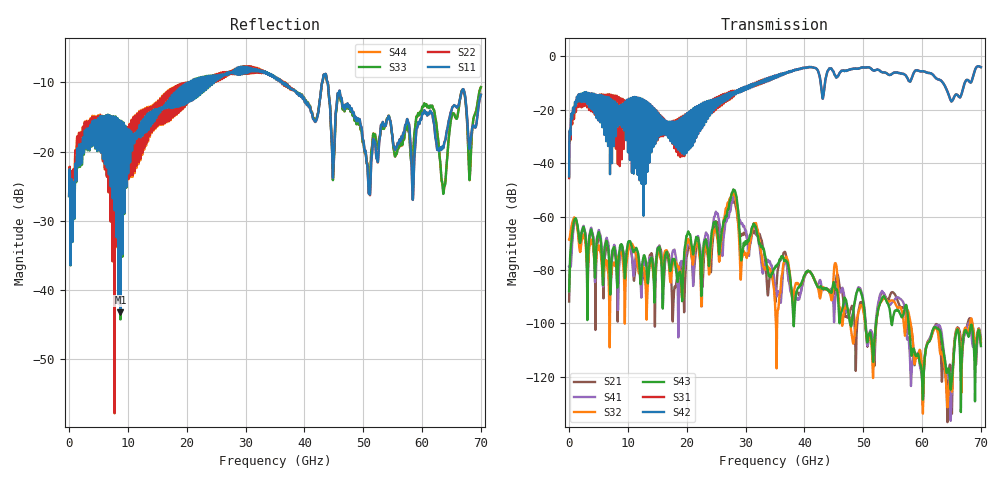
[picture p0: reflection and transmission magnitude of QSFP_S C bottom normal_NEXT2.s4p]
! AWR Design Environment (8415) Tue Jan 08 12:00:01 2019
! Document = 'QSFP Channel_S'
! nPorts: 4, nXvals: 7001
# HZ S DB R 50
!Freq DBS11 AngS11 DBS12 AngS12 DBS13 AngS13 DBS14 AngS14
!	DBS21 AngS21 DBS22 AngS22 DBS23 AngS23 DBS24 AngS24
!	DBS31 AngS31 DBS32 AngS32 DBS33 AngS33 DBS34 AngS34
!	DBS41 AngS41 DBS42 AngS42 DBS43 AngS43 DBS44 AngS44
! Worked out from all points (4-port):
!   7000 points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, 10 MHz to 70 GHz, reference 50 ohm
!   strongest paths, dB at 10 MHz, 17.51 GHz, 35.01 GHz, 52.51 GHz, 70 GHz:
!     S42: -44.9, -29.9, -7.3, -5.0, -4.0
!     S31: -45.6, -27.8, -7.4, -5.0, -4.0
!     S43: -88.0, -76.9, -79.1, -94.9, -108.5
!     S32: -68.7, -79.6, -92.6, -95.2, -106.9
!     S41: -78.7, -74.4, -85.9, -92.7, -107.5
!     S21: -91.8, -91.3, -91.2, -93.8, -105.6
!   lowest |S11| = -43.2 dB at 8.73 GHz (marker M1), VSWR 1.01, Z = 49.5 - j0.488 ohm
!   |S11| at or under -10 dB: start of sweep to 20.43 GHz; 36.44 GHz to 43.04 GHz (6.602 GHz wide, 16.6 % of centre); 43.96 GHz to end of sweep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
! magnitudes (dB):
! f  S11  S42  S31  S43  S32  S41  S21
! 10 MHz  -26.4  -44.9  -45.6  -88.0  -68.7  -78.7  -91.8
! 1.63 GHz  -20.1  -14.2  -15.6  -66.9  -69.1  -67.9  -67.3
! 8.73 GHz  -43.2  -21.2  -17.0  -70.6  -73.1  -72.3  -72.8
! 22.51 GHz  -10.0  -19.1  -19.6  -87.6  -91.6  -86.2  -78.4
! 27.87 GHz  -8.5  -13.6  -13.9  -50.2  -51.2  -53.1  -53.8
! 34.07 GHz  -8.8  -8.8  -8.9  -82.0  -79.4  -76.7  -83.1
! 70 GHz  -11.8  -4.0  -4.0  -108.5  -106.9  -107.5  -105.6
